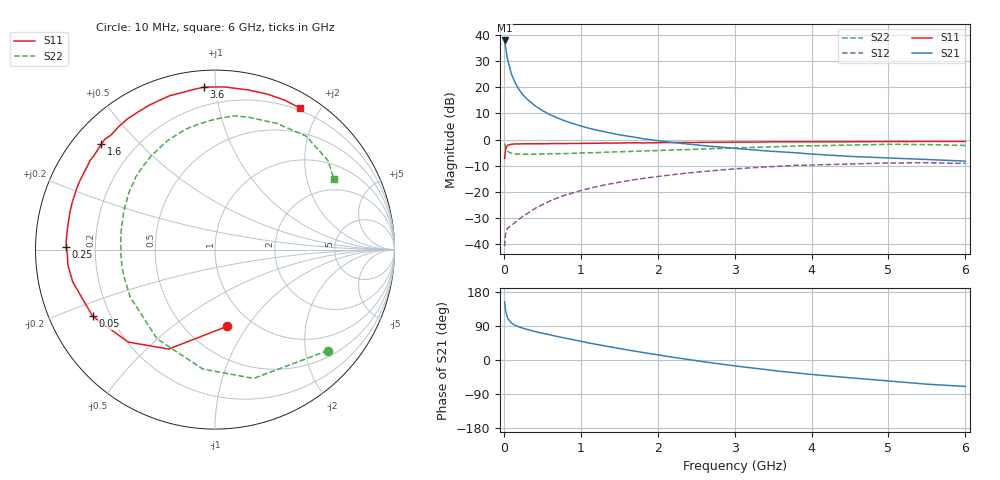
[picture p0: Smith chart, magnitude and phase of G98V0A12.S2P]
! SIEMENS Small Signal Semiconductors
! BFG235
! Si NPN RF Bipolar Junction Transistor in SOT223
! VCE = 8 V  IC = 120 mA
! Common Emitter S-Parameters:  July  1994
# GHz  S  MA  R  50
!  f  S11  S21  S12  S22
! GHz  MAG  ANG  MAG  ANG  MAG  ANG  MAG  ANG
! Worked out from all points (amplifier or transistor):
!   40 points, 10 MHz to 6 GHz, reference 50 ohm
!   highest |S21| = 37.8 dB at 10 MHz (marker M1)
!   |S21| within 3 dB of that: start of sweep to 25.17 MHz
!   unconditionally stable (mu >= 1): 468.9 MHz to 1.485 GHz
!   at 200 MHz: K = 0.79, MSG = 24.7 dB, |S12| = -30.4 dB
!   at 1.5 GHz: K = 1.00, MSG = 9.1 dB, |S12| = -16.3 dB
!   at 6 GHz: K = 0.88, MSG = 0.4 dB, |S12| = -9.1 dB
!   S11 on the Smith chart (normalised r, x): 10 MHz: 0.77, -0.81; 50 MHz: 0.13, -0.25; 250 MHz: 0.09, +0.01; 1.6 GHz: 0.08, +0.39; 3.6 GHz: 0.09, +0.93; 6 GHz: 0.17, +1.75
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0.01  0.4334 -81.3  77.95 153.5  0.0092 64.6  0.8437 -41.8
0.02  0.6114 -115.0  62.23 134.9  0.0148 49.8  0.7493 -73.3
0.03  0.7067 -133.2  49.32 123.1  0.0179 42.3  0.6689 -95.8
0.05  0.7764 -151.4  33.15 110.1  0.0203 34.3  0.5926 -123.0
0.1  0.8128 -167.2  17.56 97.5  0.0232 35.4  0.5414 -150.8
0.15  0.8244 -174.2  11.83 91.3  0.0264 41.6  0.5291 -162.7
0.2  0.8228 -177.8  8.853 87.2  0.0303 46.1  0.5275 -169.2
0.25  0.8288 178.9  7.133 83.7  0.0344 49.5  0.5245 -173.7
0.3  0.8306 176.6  5.955 80.9  0.0383 52.1  0.5248 -177.4
0.4  0.8303 171.8  4.484 75.5  0.0479 55.3  0.5248 177.3
0.5  0.8316 168.3  3.578 70.7  0.0571 56.9  0.5289 173.1
0.6  0.8353 164.9  2.987 66.5  0.0671 57.1  0.5325 169.2
0.7  0.8382 161.3  2.574 61.8  0.0772 56.9  0.537 165.8
0.9  0.8428 156.0  2.014 53.5  0.0962 54.6  0.5455 159.7
1.1  0.8469 149.5  1.652 45.1  0.1157 51.6  0.5577 153.7
1.6  0.8641 137.1  1.168 27.0  0.1622 41.8  0.5883 140.1
2.2  0.8767 123.7  0.878 7.2  0.2137 28.9  0.6322 124.2
3.2  0.8937 102.2  0.642 -20.4  0.2875 5.8  0.7035 98.1
3.6  0.9069 94.0  0.582 -30.1  0.3105 -4.1  0.7352 87.0
4.5  0.9088 78.3  0.477 -46.9  0.3408 -24.1  0.7833 63.8
5.5  0.9186 65.0  0.416 -63.8  0.3601 -46.2  0.8015 38.3
6  0.9198 59.0  0.387 -69.8  0.3499 -54.7  0.7709 30.7
